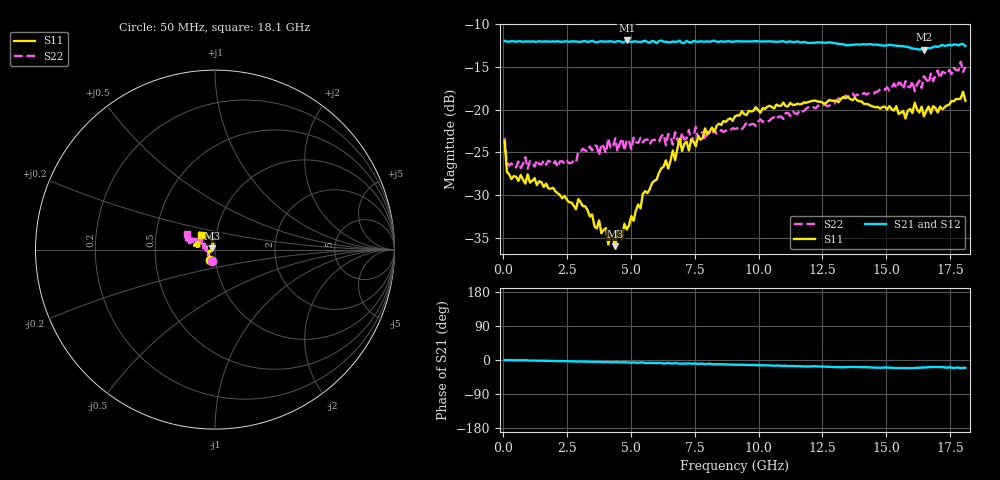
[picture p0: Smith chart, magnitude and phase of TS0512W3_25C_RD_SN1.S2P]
! Network Analyzer HP8720D.06.14 Serial No. US36140669
! 17 Jun 2005  08:11:53
! Frequency  S11  S21  S12  S22
# HZ  S  DB R 50
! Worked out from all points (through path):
!   201 points, 50 MHz to 18.1 GHz, reference 50 ohm
!   highest |S21| = -11.88 dB at 4.833 GHz (marker M1); lowest = -13.0 dB at 16.48 GHz (marker M2)
!   group delay of S21, straight-line fit = 3.5 ps
!   lowest |S11| = -36.0 dB at 4.382 GHz (marker M3), VSWR 1.03, Z = 48.6 + j0.717 ohm
!   |S11| at or under -10 dB: start of sweep to end of sweep
!   |S22| runs from -26.9 to -14.4 dB; largest |S21 - S12| = 0.0072
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5e7  -23.63 -117.0  -11.93 -0.2  -11.96 -0.2  -23.30 -104.4
1.4025e8  -27.27 -139.9  -12.02 -0.3  -11.99 -0.2  -26.18 -145.1
3.2075e8  -28.12 -155.3  -11.97 -0.6  -11.98 -0.5  -26.27 -163.4
2.12575e9  -29.76 -161.3  -11.97 -3.0  -12.02 -2.9  -26.71 168.6
3.1185e9  -31.29 -165.4  -11.97 -4.1  -12.02 -4.3  -24.57 171.2
3.75025e9  -32.96 -177.0  -12.02 -4.3  -12.07 -4.3  -25.35 168.5
4.382e9  -35.98 152.3  -12.06 -5.3  -11.98 -5.8  -23.34 168.0
4.47225e9  -34.11 143.1  -11.96 -5.8  -12.01 -5.4  -24.91 171.1
4.83325e9  -34.03 137.5  -11.88 -6.1  -11.87 -6.8  -23.50 160.9
6.09675e9  -27.41 105.9  -11.96 -7.7  -11.90 -7.7  -23.79 161.6
6.63825e9  -24.78 107.7  -12.01 -9.3  -12.08 -8.8  -24.10 155.3
6.7285e9  -25.92 109.0  -12.05 -7.8  -12.13 -8.6  -22.63 155.7
6.909e9  -23.36 107.4  -11.91 -10.1  -12.05 -9.6  -24.22 152.1
7.27e9  -24.79 104.3  -12.07 -9.0  -12.07 -9.9  -22.36 154.4
7.36025e9  -23.45 102.0  -12.13 -9.8  -12.09 -9.2  -23.82 157.2
7.54075e9  -24.28 103.7  -11.99 -9.3  -11.90 -10.3  -22.03 156.6
7.90175e9  -22.17 112.4  -12.03 -11.0  -12.01 -10.5  -23.52 150.1
9.075e9  -20.76 124.3  -11.99 -12.2  -11.99 -12.1  -22.25 147.0
1.21435e10  -18.93 160.1  -12.15 -16.3  -12.13 -16.4  -19.71 147.8
1.512175e10  -19.57 167.4  -12.39 -20.1  -12.38 -19.7  -17.75 158.6
1.64755e10  -20.78 159.7  -12.95 -19.4  -12.88 -19.1  -16.06 158.3
1.81e10  -18.96 132.5  -12.54 -20.7  -12.58 -22.3  -14.98 151.2
